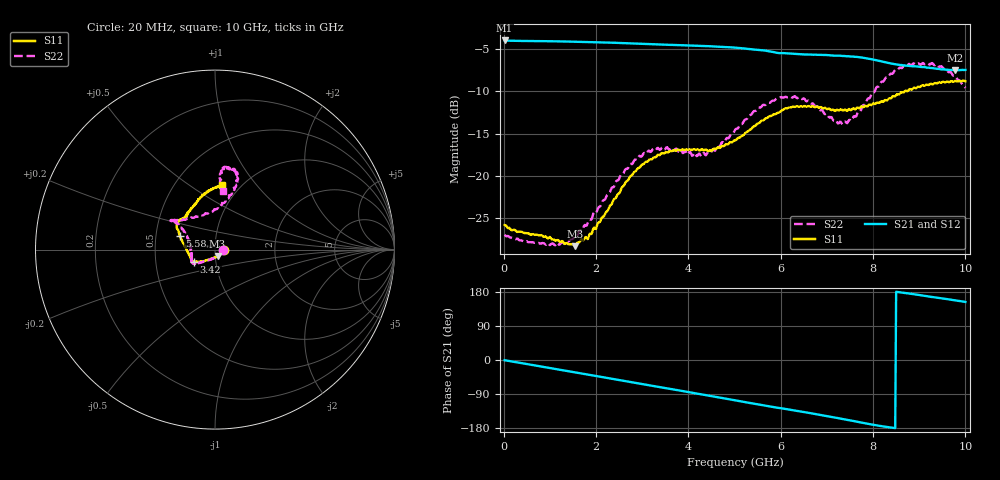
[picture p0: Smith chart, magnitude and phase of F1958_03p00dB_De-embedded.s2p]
! Integrated Device Technology
! Corporate Headquarters
! 6024 Silver Creek Valley Road
! San Jose, CA 95138  USA
! Phone:  1-408-284-8200
! Toll Free:  1-800-223-1366
! Webpage:  http://www.idt.com/
! Timing and RF Division
! 515 Groton Road, Suite 102
! Westford, MA 01886-6024
! Device:  F1958
! Description: 7-bit 0.25 dB Digital Step Attenuator
! Frequency:  0.001 -  6.000 GHz
! Package:  4x4 mm Thin QFN Plastic Package: 24 pin
! Ports:  2 RF, 12 DC
!  Pin  1  = D0
!  Pin  2  = VDD
!  Pin  3  = VMODE
!  Pin  4  = GND
!  Pin  5  = RF1  =  Port 1
!  Pin  6  = GND
!  Pin  7  = GND
!  Pin  8  = GND
!  Pin  9  = GND
!  Pin 10  = GND
!  Pin 11  = GND
!  Pin 12  = GND
!  Pin 13  = GND
!  Pin 14  = RF2  =  Port 2
!  Pin 15  = GND
!  Pin 16  = LE
!  Pin 17  = CLK
!  Pin 18  = DATA
!  Pin 19  = D6
!  Pin 20  = D5
!  Pin 21  = D4
!  Pin 22  = D3
!  Pin 23  = D2
!  Pin 24  = D1
! State:  12
! Atten State:  3.00 dB
! Voltage:  +3.30 Volts
! Current:  0.258 mA
! Data:  The device was measured on a F1958 evaluation board which has
!  individual transmission lines to the RF pins.  Data was collected
!  using a calibrated network analyzer.  The evaluation board was
!  de-embedded using Automatic Fixture Removal (AFR).
!  The reference plane is the edge of the package pin.
! Misc:
!  Action Tracker AT0419
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# GHz S dB R 50
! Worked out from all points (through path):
!   500 points, 20 MHz to 10 GHz, reference 50 ohm
!   highest |S21| = -4.00 dB at 20 MHz (marker M1); lowest = -7.5 dB at 9.78 GHz (marker M2)
!   group delay of S21, straight-line fit = 58.3 ps
!   lowest |S11| = -28.3 dB at 1.54 GHz (marker M3), VSWR 1.08, Z = 51.3 - j3.68 ohm
!   |S11| at or under -10 dB: start of sweep to 8.685 GHz
!   |S22| runs from -28.1 to -6.6 dB; largest |S21 - S12| = 0.0018
!   S11 on the Smith chart (normalised r, x): 20 MHz: 1.11, -0.00; 3.42 GHz: 0.78, -0.11; 5.58 GHz: 0.66, +0.11; 10 GHz: 0.83, +0.69
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0.02  -25.77 -2.5  -4.00 -0.6  -4.00 -0.5  -26.92 -3.0
0.96  -27.35 -29.7  -4.09 -20.3  -4.08 -20.3  -27.90 -41.3
1.54  -28.27 -68.0  -4.15 -32.6  -4.14 -32.5  -27.08 -85.6
1.7  -27.47 -80.4  -4.16 -35.9  -4.16 -35.8  -26.45 -97.9
1.86  -26.84 -94.1  -4.18 -39.3  -4.18 -39.3  -25.12 -106.3
2.72  -20.21 -137.8  -4.33 -57.5  -4.32 -57.5  -18.76 -140.6
3.36  -17.51 -148.3  -4.48 -71.1  -4.48 -71.2  -16.78 -148.5
3.42  -17.29 -149.4  -4.49 -72.3  -4.50 -72.4  -16.67 -151.3
4.34  -16.96 -161.4  -4.64 -91.8  -4.66 -91.8  -17.28 -179.3
4.6  -16.80 -167.2  -4.72 -97.3  -4.73 -97.3  -16.78 165.9
5.02  -15.78 176.9  -4.85 -106.5  -4.86 -106.5  -14.47 151.6
5.58  -13.47 158.5  -5.16 -118.7  -5.17 -118.7  -11.82 144.9
6.16  -11.95 147.6  -5.52 -130.4  -5.53 -130.3  -10.72 146.2
6.68  -11.76 140.7  -5.67 -141.0  -5.69 -140.9  -11.44 141.9
7.22  -12.16 135.2  -5.80 -152.9  -5.81 -152.7  -13.61 118.7
7.46  -12.18 130.7  -5.86 -158.3  -5.87 -158.2  -13.58 98.6
7.96  -11.63 120.3  -6.21 -170.0  -6.21 -170.0  -10.38 74.9
8.34  -10.85 110.4  -6.65 -177.5  -6.66 -177.6  -8.24 71.6
8.72  -9.93 100.8  -6.98 176.4  -6.97 176.5  -7.06 75.1
9.16  -9.21 90.2  -7.20 168.5  -7.18 168.5  -6.68 81.5
9.78  -8.77 83.8  -7.51 157.6  -7.53 157.6  -8.18 85.3
10  -8.79 83.6  -7.47 153.2  -7.50 153.3  -9.59 82.3
